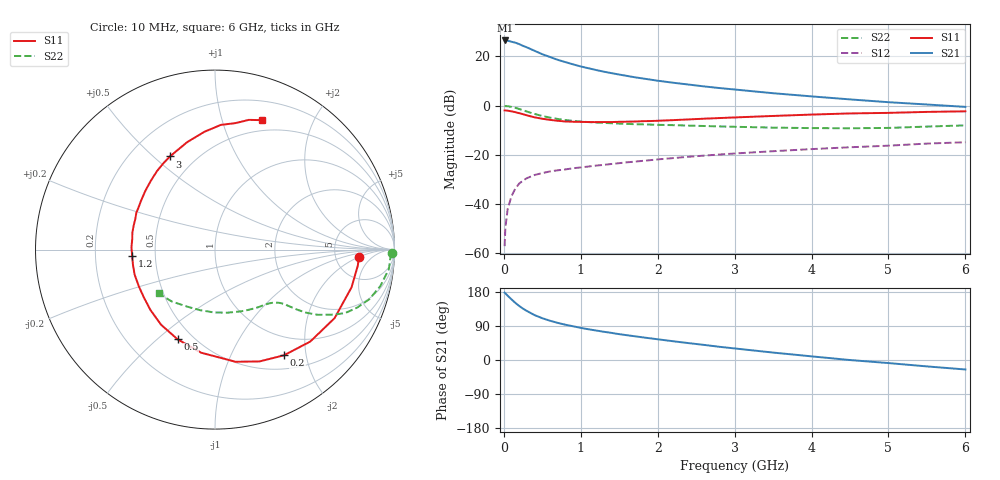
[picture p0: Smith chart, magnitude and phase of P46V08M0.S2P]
! SIEMENS Small Signal Semiconductors
! BFP182
! Si NPN RF Bipolar Junction Transistor in SOT143
! VCE = 6 V  IC = 8 mA
! Common Emitter S-Parameters:  March  1996
# GHz  S  MA  R  50
!  f  S11  S21  S12  S22
! GHz  MAG  ANG  MAG  ANG  MAG  ANG  MAG  ANG
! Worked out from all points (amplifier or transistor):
!   36 points, 10 MHz to 6 GHz, reference 50 ohm
!   highest |S21| = 26.5 dB at 20 MHz (marker M1)
!   |S21| within 3 dB of that: start of sweep to 313.3 MHz
!   unconditionally stable (mu >= 1): 1.364 GHz to 5.476 GHz
!   at 250 MHz: K = 0.27, MSG = 27.3 dB, |S12| = -30.4 dB
!   at 1.4 GHz: K = 1.01, MAG = 17.8 dB, |S12| = -23.7 dB
!   at 6 GHz: K = 0.95, MSG = 7.2 dB, |S12| = -14.9 dB
!   lowest NFmin = 1.40 dB at 450 MHz
!   S11 on the Smith chart (normalised r, x): 10 MHz: 8.69, -1.91; 200 MHz: 0.70, -1.62; 500 MHz: 0.41, -0.58; 1.2 GHz: 0.37, -0.03; 3 GHz: 0.36, +0.57; 6 GHz: 0.39, +1.36
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0.01  0.8023 -2.8  20.91 177.7  0.0014 86.7  0.9853 -1.2
0.02  0.8009 -6.3  21.11 176.0  0.0033 91.9  0.9784 -2.5
0.05  0.7895 -15.4  20.88 169.6  0.008 85.5  0.9748 -6.4
0.1  0.768 -29.8  19.87 159.9  0.0146 74.1  0.9436 -12.4
0.15  0.7377 -44.0  19.02 150.7  0.0208 68.3  0.9036 -17.8
0.2  0.7032 -56.8  17.79 142.5  0.0262 63.0  0.8554 -22.2
0.25  0.6706 -68.3  16.39 135.4  0.0302 58.7  0.808 -25.9
0.3  0.6354 -79.6  15.27 129.3  0.0337 54.1  0.7587 -28.5
0.4  0.5798 -97.6  13.01 118.4  0.0391 49.8  0.6783 -32.4
0.5  0.5416 -112.6  11.09 110.3  0.0427 45.7  0.6169 -34.7
0.6  0.5154 -125.6  9.742 103.6  0.0462 44.0  0.5728 -36.0
0.7  0.4926 -136.9  8.535 98.0  0.0487 42.5  0.5372 -36.9
0.9  0.4712 -154.2  6.907 89.0  0.0536 41.4  0.4909 -38.2
1.1  0.4649 -169.4  5.756 81.1  0.0581 40.8  0.4645 -39.7
1.2  0.463 -175.8  5.294 77.8  0.0606 40.6  0.4548 -40.6
1.7  0.476 158.8  3.78 62.7  0.0729 41.1  0.4206 -45.8
2.2  0.5084 139.6  2.925 49.5  0.0861 39.8  0.4017 -53.0
3  0.5766 115.8  2.13 30.5  0.1068 35.8  0.3724 -67.7
3.5  0.6181 104.6  1.79 19.6  0.1188 32.5  0.3582 -78.7
4.5  0.6956 87.3  1.341 -0.1  0.1429 25.8  0.3475 -103.7
5.5  0.747 75.4  1.056 -16.9  0.1697 19.3  0.376 -129.7
6  0.7678 69.9  0.945 -25.0  0.1809 14.8  0.3983 -142.2
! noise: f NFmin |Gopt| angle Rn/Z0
0.45  1.4  0.26  41  0.29
0.9  1.5  0.25  83  0.23
1.8  2  0.21  162  0.2
